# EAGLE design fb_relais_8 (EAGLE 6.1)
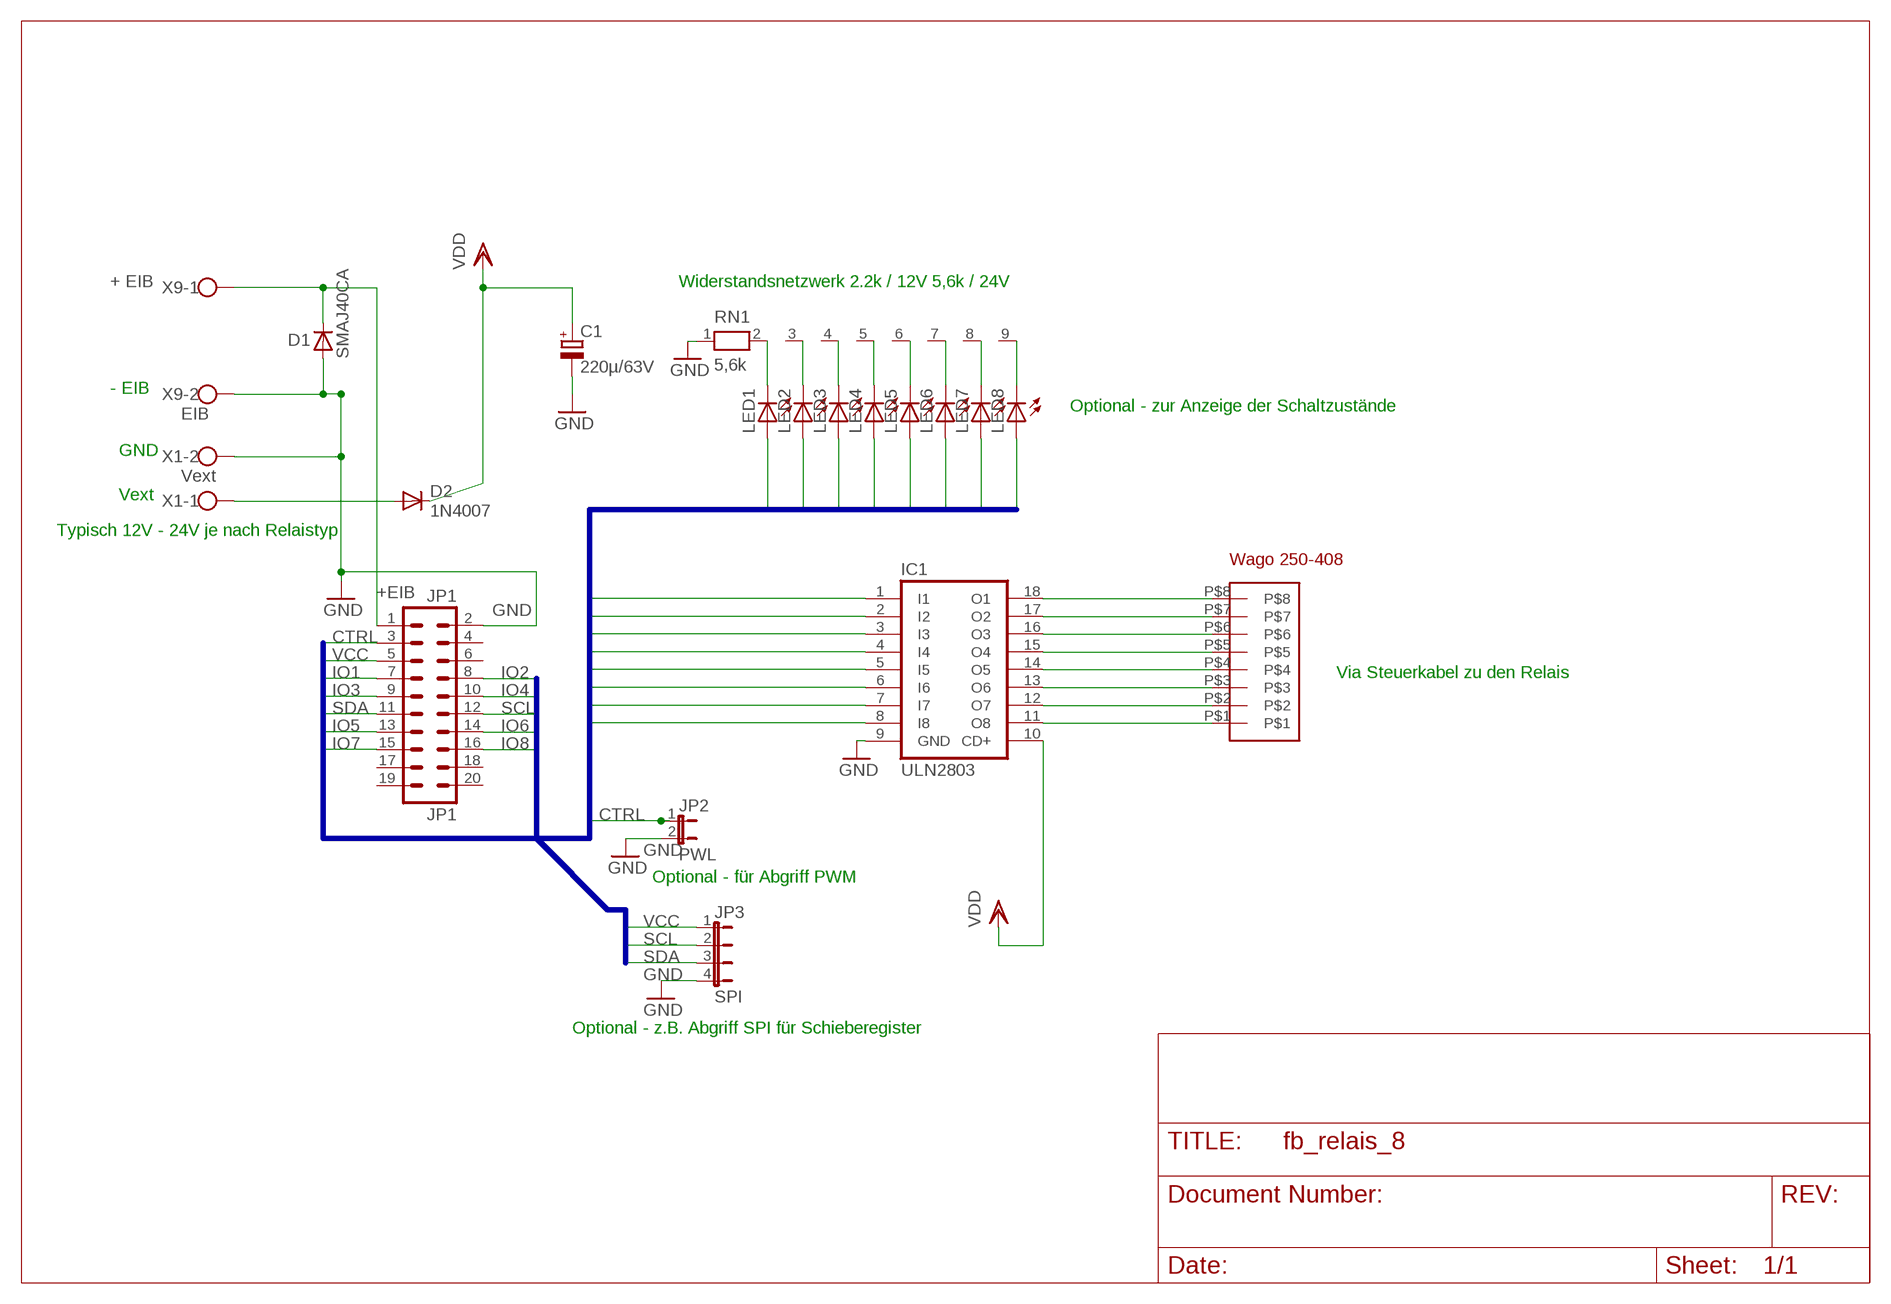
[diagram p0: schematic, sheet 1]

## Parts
C1  220µ/63V  CPOL-EUE5-10.5  [E5-10,5]
D1  SMAJ40CA  D-SMB  [SMB]
D2  1N4007  1N4004STEHEND  [RAD2,5]
IC1  ULN2803  ULN2803A  [DIL18]
JP1  JP1  ML20  [ML20]
JP2  PWL  JP1E  [JP1]
JP3  SPI  JP4E  [JP4]
LED1  TLLG4400  [LED3MM]
LED2  TLLG4400  [LED3MM]
LED3  TLLG4400  [LED3MM]
LED4  TLLG4400  [LED3MM]
LED5  TLLG4400  [LED3MM]
LED6  TLLG4400  [LED3MM]
LED7  TLLG4400  [LED3MM]
LED8  TLLG4400  [LED3MM]
RN1  5,6k  RN08  [RN-9]
U$1  WAGO205-408  [WAGO250-408]
X1  Vext  W237-102  [W237-102]
X9  EIB  W237-102  [W237-102]

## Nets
+EIB: D1.1(C) JP1.1 X9.1
CTRL: JP1.3 JP2.1
GND: C1.- D1.2(A) IC1.9(GND) JP1.2 JP2.2 JP3.4 RN1.1 X1.2 X9.2
IO1: IC1.8(I8) JP1.7 LED1.A
IO2: IC1.7(I7) JP1.8 LED2.A
IO3: IC1.6(I6) JP1.9 LED3.A
IO4: IC1.5(I5) JP1.10 LED4.A
IO5: IC1.4(I4) JP1.13 LED5.A
IO6: IC1.3(I3) JP1.14 LED6.A
IO7: IC1.2(I2) JP1.15 LED7.A
IO8: IC1.1(I1) JP1.16 LED8.A
N$1: IC1.11(O8) U$1.P$1
N$2: IC1.12(O7) U$1.P$2
N$3: IC1.13(O6) U$1.P$3
N$4: IC1.14(O5) U$1.P$4
N$5: IC1.15(O4) U$1.P$5
N$6: IC1.16(O3) U$1.P$6
N$7: IC1.17(O2) U$1.P$7
N$8: IC1.18(O1) U$1.P$8
N$9: LED1.K(C) RN1.2
N$10: LED3.K(C) RN1.4
N$11: LED4.K(C) RN1.5
N$12: LED5.K(C) RN1.6
N$13: LED6.K(C) RN1.7
N$14: LED7.K(C) RN1.8
N$15: LED8.K(C) RN1.9
N$16: LED2.K(C) RN1.3
N$17: D2.A X1.1
SCL: JP1.12 JP3.2
SDA: JP1.11 JP3.3
VCC: JP1.5 JP3.1
VDD: C1.+ D2.C IC1.10(CD+)
Unconnected: JP1.4 JP1.6 JP1.17 JP1.18 JP1.19 JP1.20

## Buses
IO[1..8],CTRL,SDA,SCL,VCC

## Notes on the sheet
- + EIB | Widerstandsnetzwerk 2.2k / 12V 5,6k / 24V
- - EIB
- Optional - zur Anzeige der Schaltzustände
- GND
- Vext
- Typisch 12V - 24V je nach Relaistyp
- Via Steuerkabel zu den Relais
- Optional - für Abgriff PWM
- Optional - z.B. Abgriff SPI für Schieberegister

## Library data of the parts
C1 = rcl:CPOL-EU: POLARIZED CAPACITOR, European symbol
D1 = semicon-smd-ipc:D-: DIODE
D2 = diode:1N4004: DIODE
IC1 = uln-udn:ULN2803A: DRIVER ARRAY
JP1 = con-harting-ml:ML20: HARTING
JP2 = jumper:JP1E: JUMPER
JP3 = jumper:JP4E: JUMPER
LED1-LED8 = led:TLLG4400: Low Current (2mA) LED 3 mm Tinted Diffused Package color GREEN; MF: VISHAY SEMICONDUCTOR; OC_FARNELL: 1612435
RN1 = resistor-net:RN08: RESISTOR NETWORK; OC_FARNELL: unknown; OC_NEWARK: unknown
U$1 = wago-250er:WAGO205-408
X1 X9 = con-wago-500:W237-102: WAGO SCREW CLAMP; MPN: 237-102; OC_FARNELL: unknown; OC_NEWARK: 70K9898

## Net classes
0 SELV: width 0.406 mm
1 230Vac: width 1.93 mm, clearance 5.08 mm to class 0, clearance 1.905 mm

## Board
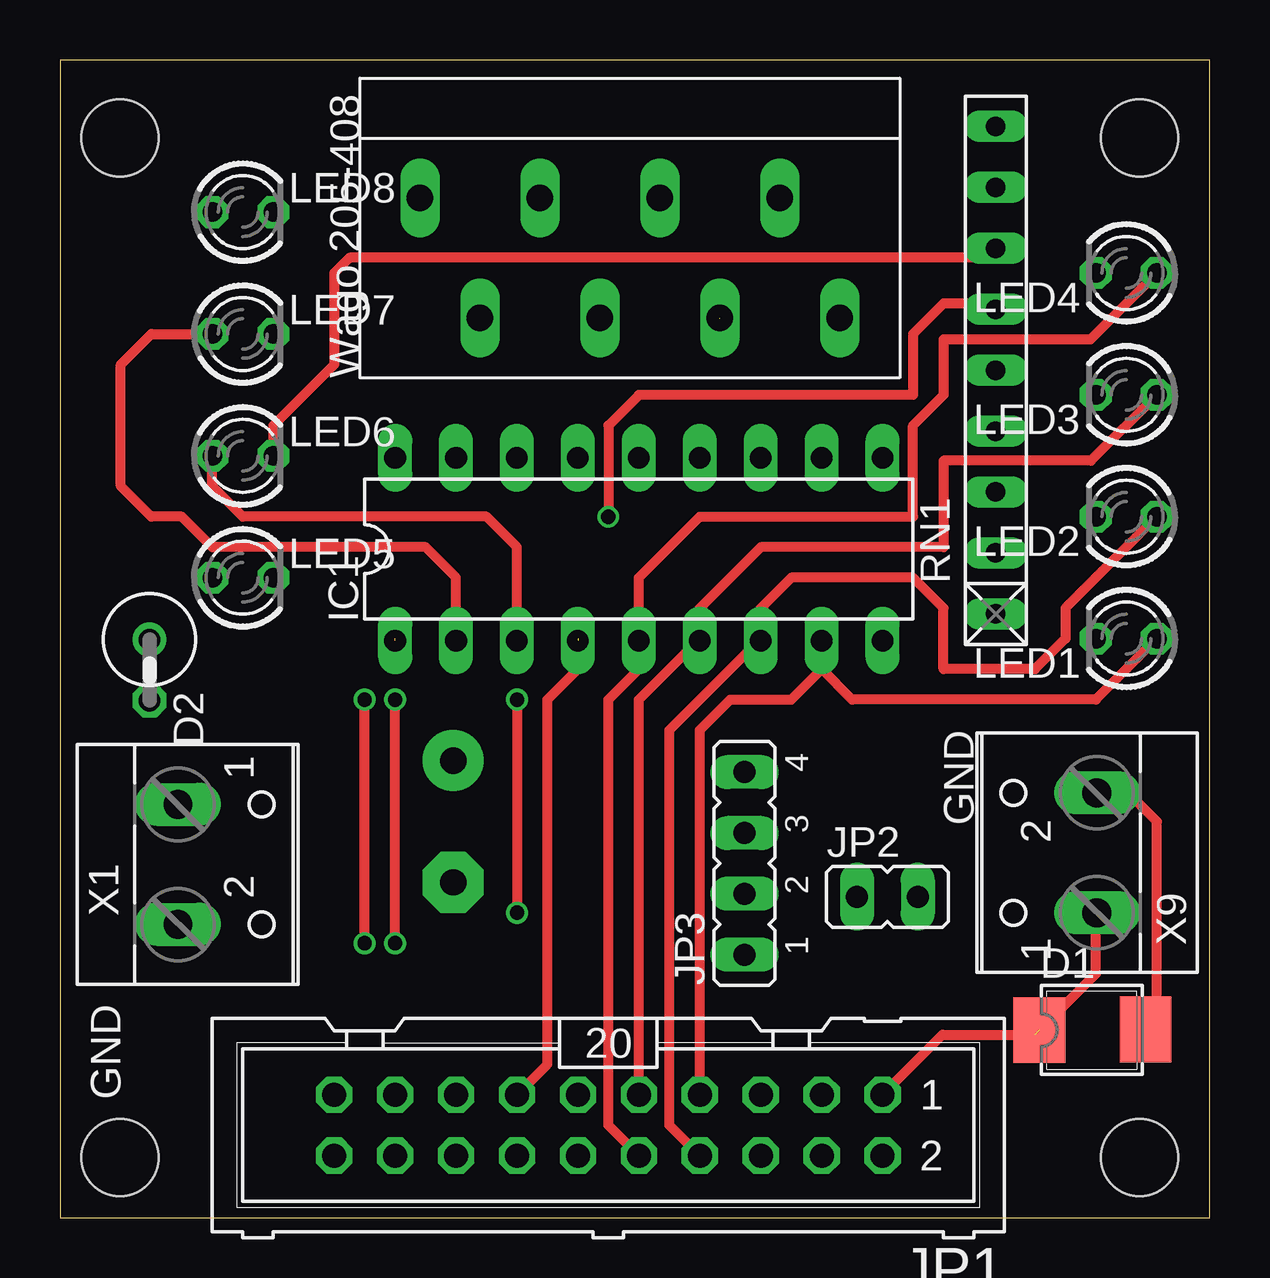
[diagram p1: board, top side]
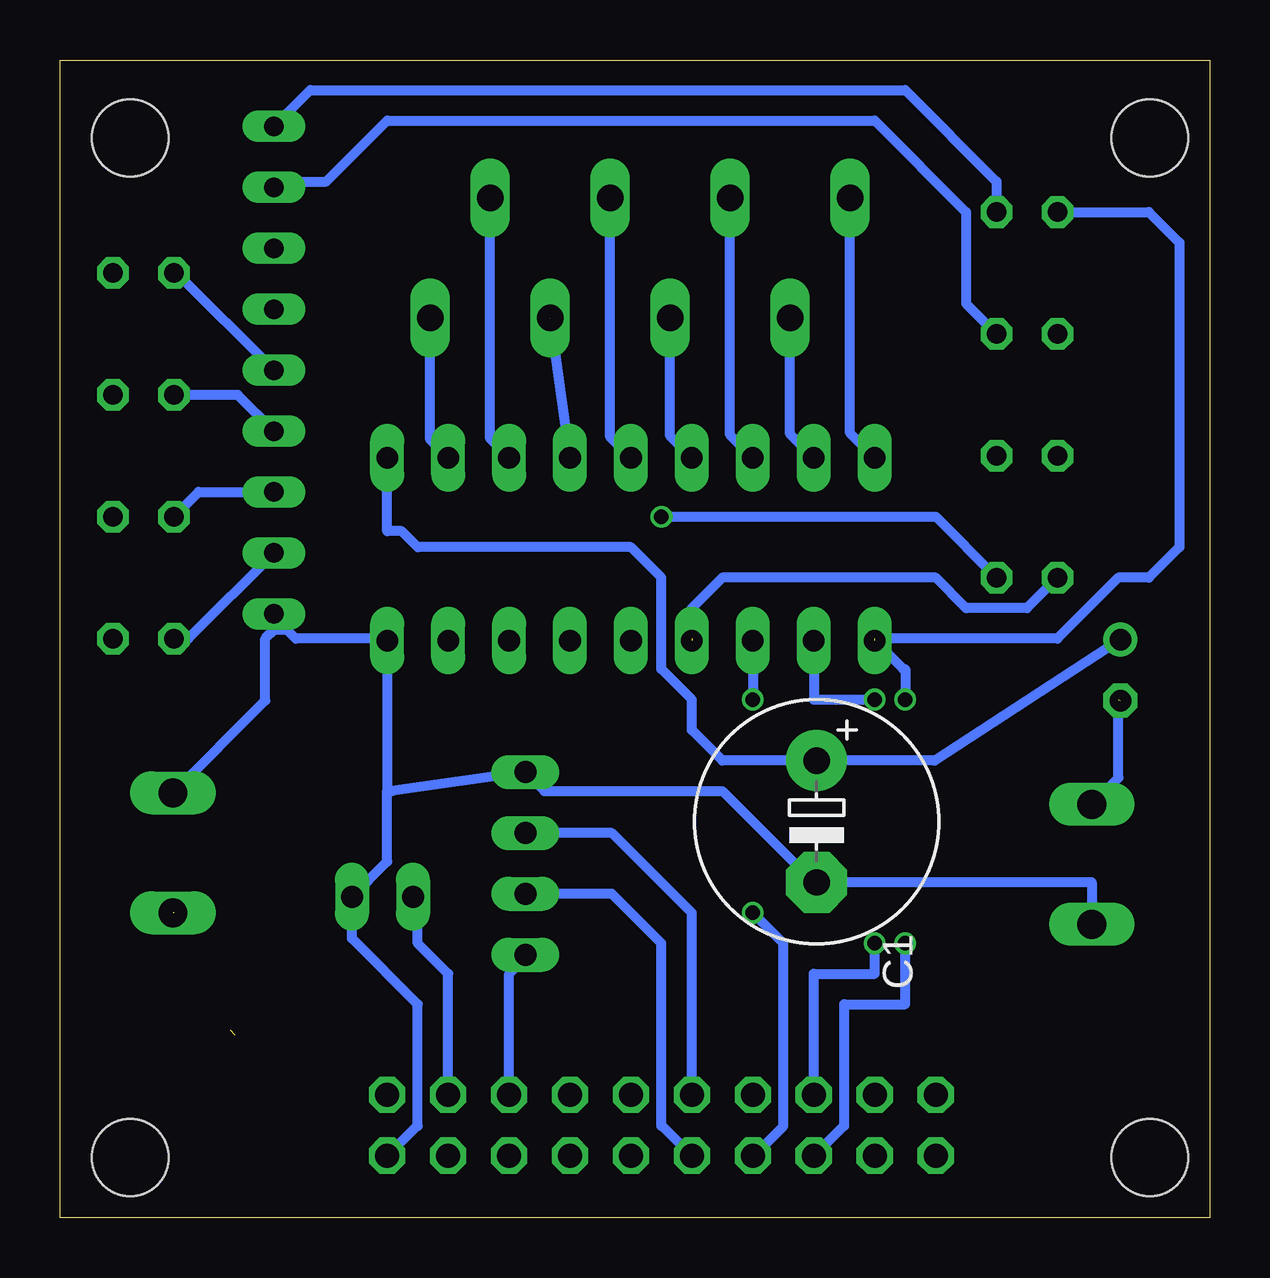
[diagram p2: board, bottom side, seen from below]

Size 47.93 x 48.25 mm. Coordinates in mm from the lower left corner, seen from the top.
Outline: 0,0 47.93,0 47.93,48.25 0,48.25 0,0
Copper layers (1*16): Top 0.035mm / dielectric 1.5mm / Bottom 0.035mm
Design rules: minimum track width 6mil, minimum drill 12mil, track to track 6mil, track to pad 6mil, pad to pad 6mil, via to via 6mil, smd to smd 0mil, copper to edge 10mil, drill to drill 10mil, minimum pad ring 10mil, minimum via ring 6mil, stop-mask expansion 2mil, vias tented up to drill 100mil, thermal gap 10mil
Holes 3.2 mm at 45,2.5 2.5,2.5 45,45 2.5,45

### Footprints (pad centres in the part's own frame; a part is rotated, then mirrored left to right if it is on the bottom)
E5-10,5 = drill 1.1 pad 2.54: + -2.54,0 | drill 1.1 pad 2.54 octagon: - 2.54,0
SMB = smd 2.159 x 2.743: 1 -2.311,-0.127; 2 2.108,-0.102
RAD2,5 = drill 0.9 octagon: A 1.27,0 | drill 0.9: C -1.27,0
DIL18 = drill 0.9 long: 1 -10.16,-3.81; 2 -7.62,-3.81; 3 -5.08,-3.81; 4 -2.54,-3.81; 5 0,-3.81; 6 2.54,-3.81; 7 5.08,-3.81; 8 7.62,-3.81; 9 10.16,-3.81; 10 10.16,3.81; 11 7.62,3.81; 12 5.08,3.81; 13 2.54,3.81; 14 0,3.81; 15 -2.54,3.81; 16 -5.08,3.81; 17 -7.62,3.81; 18 -10.16,3.81
ML20 = drill 1 octagon: 1 -11.43,-1.27; 2 -11.43,1.27; 3 -8.89,-1.27; 4 -8.89,1.27; 5 -6.35,-1.27; 6 -6.35,1.27; 7 -3.81,-1.27; 8 -3.81,1.27; 9 -1.27,-1.27; 10 -1.27,1.27; 11 1.27,-1.27; 12 1.27,1.27; 13 3.81,-1.27; 14 3.81,1.27; 15 6.35,-1.27; 16 6.35,1.27; 17 8.89,-1.27; 18 8.89,1.27; 19 11.43,-1.27; 20 11.43,1.27
JP1 = drill 0.914 long: 1 0,-1.27; 2 0,1.27
JP4 = drill 0.914 long: 1 -3.81,0; 2 -1.27,0; 3 1.27,0; 4 3.81,0
LED3MM = drill 0.813 octagon: A -1.27,0; K 1.27,0
RN-9 = drill 0.813 long: 1 -10.16,0; 2 -7.62,0; 3 -5.08,0; 4 -2.54,0; 5 0,0; 6 2.54,0; 7 5.08,0; 8 7.62,0; 9 10.16,0
WAGO250-408 = drill 1.1 long: P$1 0,0; P$2 5,2.5; P$3 0,5; P$4 5,7.5; P$5 0,10; P$6 5,12.5; P$7 0,15; P$8 5,17.5
W237-102 = drill 1.194 long: 1 -2.5,-1.27; 2 2.5,-1.27

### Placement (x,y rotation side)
C1  16.39,16.51 270 bottom
D1  43.14,7.94 0 top
D2  3.73,22.82 270 top
IC1  24.13,27.86 0 top
JP1  22.86,3.85 180 top
JP2  34.49,13.37 270 top
JP3  28.53,14.76 90 top
LED1  44.45,24.13 180 top
LED2  44.45,29.21 180 top
LED3  44.45,34.29 180 top
LED4  44.45,39.37 180 top
LED5  7.62,26.67 0 top
LED6  7.62,31.75 0 top
LED7  7.62,36.83 0 top
LED8  7.62,41.91 0 top
RN1  39.01,35.32 90 top
U$1  32.5,37.5 90 top
X1  6.19,14.72 270 top
X9  41.95,15.2 90 top

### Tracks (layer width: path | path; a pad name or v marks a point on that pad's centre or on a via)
+EIB  (2 unrouted)
  Top 0.406: JP1.1 36.79,7.62 40.64,7.62 43.18,10.16 43.18,12.7
CTRL
  Bottom 0.406: JP1.3 31.75,10.16 33.02,11.43 33.02,13.17 JP2.1
GND
  Top 0.406: 45.72,7.37 D1.2 45.72,8.31 45.72,16.51 44.53,17.7 X9.2
  Bottom 0.406: 34.29,17.78 34.09,17.78 JP3.4 27.74,17.78 20.32,17.78 16.51,13.97 C1.- 4.92,13.97 X1.2 | 34.29,17.78 IC1.9 34.37,24.13 38.1,24.13 38.46,24.49 39.01,24.49 | 34.29,17.78 34.29,14.84 JP2.2 35.76,11.63 33.02,8.89 33.02,3.81 33.06,3.81 JP1.2 | X9.2 39.37,21.55 39.37,24.13 39.01,24.49 | 39.01,24.49 RN1.1
IO1
  Top 0.406: JP1.7 26.67,20.32 27.94,21.59 30.48,21.59 31.75,22.86 | 31.75,22.86 IC1.8 | LED1.A 43.18,21.59 33.02,21.59 31.75,22.86
IO2
  Top 0.406: JP1.8 25.4,3.85 25.4,20.32 29.13,24.05 IC1.7 29.21,25.4 30.48,26.67 35.56,26.67 36.83,25.4 36.83,22.86 40.64,22.86 41.91,24.13 41.91,25.4 LED2.A
IO3
  Top 0.406: 26.67,24.13 26.67,25.4 29.21,27.94 36.83,27.94 36.83,31.54 36.82,31.54 42.97,31.54 LED3.A | 26.67,24.13 IC1.6 | JP1.9 24.13,21.59 26.67,24.13
IO4
  Top 0.406: JP1.10 22.86,3.85 22.86,21.59 24.13,22.86 IC1.5 24.13,26.67 26.67,29.21 35.56,29.21 35.56,33.02 36.83,34.29 36.83,36.59 36.84,36.6 42.95,36.6 LED4.A
IO5  (1 unrouted)
  Top 0.406: JP1.13 20.32,6.39 20.32,21.59 21.59,22.86 21.59,24.13
  Bottom 0.406: LED5.A 7.62,25.4 10.16,25.4 11.43,26.67 20.32,26.67 21.59,25.4 IC1.4
IO6  (via drill 0.6)
  Top 0.406: IC1.3 19.05,27.94 17.78,29.21 7.62,29.21 6.35,30.48 LED6.A | v19.05,21.59 v19.05,12.7
  Bottom 0.406: JP1.14 19.01,2.58 17.78,3.81 17.78,11.43 v19.05,12.7 | IC1.3 v19.05,21.59
IO7  (via drill 0.6)
  Top 0.406: v13.97,11.43 v13.97,21.59 | IC1.2 16.51,26.67 15.24,27.94 6.35,27.94 5.08,29.21 3.81,29.21 2.54,30.48 2.54,35.56 3.81,36.83 LED7.A
  Bottom 0.406: IC1.2 16.51,21.59 v13.97,21.59 | JP1.15 16.51,10.16 13.97,10.16 v13.97,11.43
IO8  (via drill 0.6)  (1 unrouted)
  Top 0.406: v12.7,11.43 v12.7,21.59
  Bottom 0.406: IC1.1 12.78,22.86 12.7,22.86 v12.7,21.59 | JP1.16 15.28,3.81 15.24,3.81 15.24,8.89 12.7,8.89 v12.7,11.43 | LED8.A 2.54,41.91 1.27,40.64 1.27,27.94 2.54,26.67 3.81,26.67 6.35,24.13 13.97,24.13
N$1
  Bottom 0.406: IC1.11 32.5,32.42 U$1.P$1
N$2
  Bottom 0.406: IC1.12 30,32.46 U$1.P$2
N$3  (1 unrouted)
  Bottom 0.406: IC1.13 27.48,37.5 27.5,37.52 27.49,37.48
N$4
  Bottom 0.406: IC1.14 25,32.54 U$1.P$4
N$5
  Bottom 0.406: IC1.15 22.5,32.58 U$1.P$5
N$6
  Bottom 0.406: IC1.16 20,32.62 U$1.P$6
N$7
  Bottom 0.406: IC1.17 17.5,32.66 U$1.P$7
N$8
  Bottom 0.406: IC1.18 15,32.7 U$1.P$8
N$9
  Bottom 0.406: RN1.2 42.58,24.13 LED1.K
N$10
  Bottom 0.406: RN1.4 40.52,34.29 LED3.K
N$11
  Bottom 0.406: RN1.5 43.06,39.37 LED4.K
N$12  (via drill 0.6)
  Top 0.406: RN1.6 38.77,38.1 36.83,38.1 35.56,36.83 35.56,34.29 24.13,34.29 22.86,33.02 v22.86,29.21
  Bottom 0.406: v22.86,29.21 11.43,29.21 LED5.K
N$13
  Top 0.406: RN1.7 39.01,40.01 12.06,40.01 11.43,39.37 11.43,35.56 8.89,33.02 LED6.K
N$14
  Bottom 0.406: RN1.8 38.77,43.18 36.83,43.18 34.29,45.72 13.97,45.72 10.16,41.91 10.16,38.1 LED7.K
N$15
  Bottom 0.406: RN1.9 37.5,46.99 12.7,46.99 8.89,43.18 LED8.K
N$16
  Bottom 0.406: LED2.K 42.15,30.24 RN1.3
N$17  (1 unrouted)
  Bottom 0.406: X1.1 3.81,18.33 3.81,21.59
SCL
  Bottom 0.406: JP1.12 22.82,3.81 22.86,3.81 22.86,11.43 24.92,13.49 JP3.2
SDA
  Bottom 0.406: JP1.11 21.59,12.7 24.92,16.03 JP3.3
VCC
  Bottom 0.406: JP1.5 29.21,10.16 28.53,10.84 JP3.1
VDD
  Bottom 0.406: D2.C 11.47,19.05 C1.+ 20.32,19.05 21.59,20.32 21.59,21.59 22.86,22.86 22.86,26.67 24.13,27.94 33.02,27.94 33.69,28.61 34.29,28.61 IC1.10

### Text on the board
tPlace: GND | GND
